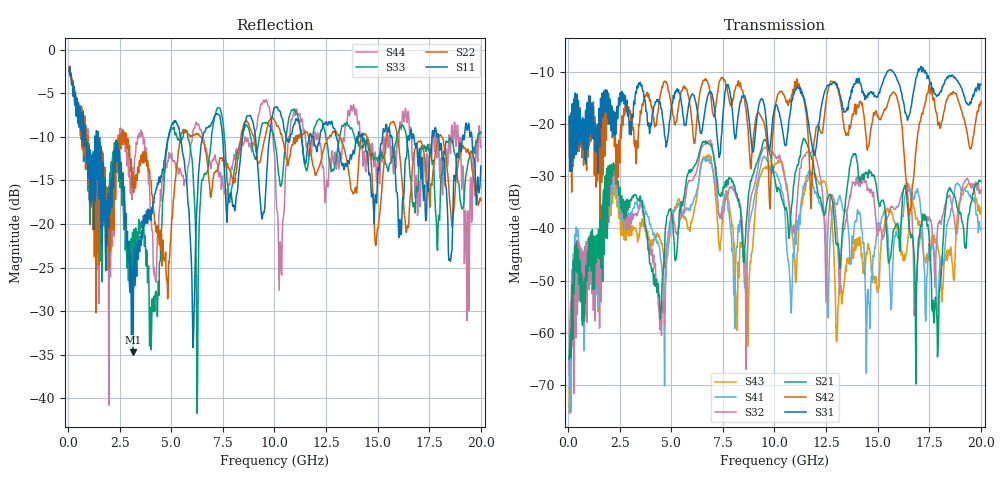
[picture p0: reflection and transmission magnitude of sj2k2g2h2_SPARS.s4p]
! FILE: E:\users\goganessyan\GBX_Backplane\FR408_backplane\1m_INBOUND_NEXT\sj2k2g2h2_SPARS.s4p
# MHZ S RI R 50.00
! FREQ  S11  S12  S13  S14
!  S21  S22  S23  S24
!  S31  S32  S33  S34
!  S41  S42  S43  S44
!  REAL  IMAG  REAL  IMAG  REAL  IMAG  REAL  IMAG
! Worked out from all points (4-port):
!   799 points, 50 MHz to 20 GHz, reference 50 ohm
!   strongest paths, dB at 50 MHz, 5.025 GHz, 10.03 GHz, 15.03 GHz, 20 GHz:
!     S31: -18.5, -16.2, -16.4, -14.4, -12.3
!     S42: -19.3, -16.6, -17.1, -18.5, -15.6
!     S21: -65.1, -37.7, -30.7, -34.7, -31.0
!     S32: -67.4, -37.3, -25.9, -40.1, -32.6
!     S41: -68.2, -38.4, -29.2, -38.9, -40.3
!     S43: -70.7, -38.7, -27.7, -51.1, -36.1
!   lowest |S11| = -34.7 dB at 3.15 GHz (marker M1), VSWR 1.04, Z = 51.2 - j1.37 ohm
!   |S11| at or under -10 dB: 1.453 GHz to 4.871 GHz (3.418 GHz wide, 108 % of centre); 5.447 GHz to 6.533 GHz (1.086 GHz wide, 18.1 % of centre); 17.95 GHz to 19.11 GHz (1.156 GHz wide, 6.24 % of centre)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
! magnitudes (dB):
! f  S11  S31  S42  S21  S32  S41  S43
! 50 MHz  -2.5  -18.5  -19.3  -65.1  -67.4  -68.2  -70.7
! 400 MHz  -7.6  -17.3  -21.2  -42.6  -44.4  -39.7  -42.9
! 3.15 GHz  -34.7  -18.7  -20.8  -34.0  -38.2  -36.1  -40.4
! 4.45 GHz  -15.2  -15.7  -14.9  -55.7  -59.4  -44.6  -42.2
! 13.88 GHz  -11.7  -12.3  -16.7  -25.9  -31.4  -39.1  -43.1
! 17.88 GHz  -10.1  -14.5  -18.1  -56.9  -41.4  -56.6  -42.8
! 20 GHz  -13.3  -12.3  -15.6  -31.0  -32.6  -40.3  -36.1
